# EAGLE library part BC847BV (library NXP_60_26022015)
NPN/NPN general-purpose transistor pair in a very small SOT363 (SC-88) Surface-Mounted Device (SMD) plastic package. AAL Eindhoven MK
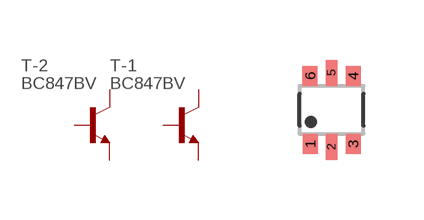
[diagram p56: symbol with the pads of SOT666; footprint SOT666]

Designator prefix T; gates -1=NPN -2=NPN

## BC847BV, BC847BV/S500, BC847BVN  [SOT666]
1  -1:E  pas
2  -1:B  pas
3  -2:C  pas
4  -2:E  pas
5  -2:B  pas
6  -1:C  pas

## Footprint SOT666 (pad centres in mm)
SOT 666 Reflow soldering foorprint Source: Philips - BAS70_1PS7XSB70_SER_8.pdf
smd 0.375 x 0.5: 1 -0.537,-0.85; 3 0.538,-0.85; 4 0.538,0.85; 6 -0.538,0.85
smd 0.3 x 0.65: 2 0,-0.925; 5 0,0.925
